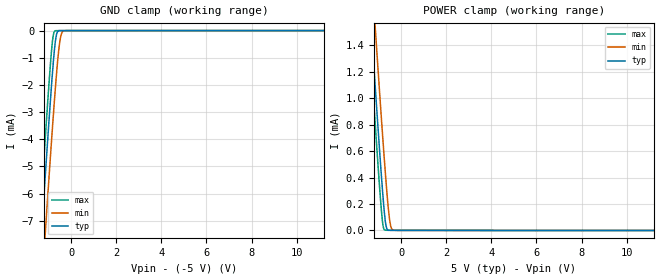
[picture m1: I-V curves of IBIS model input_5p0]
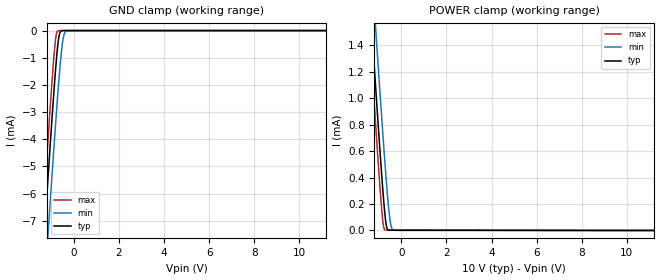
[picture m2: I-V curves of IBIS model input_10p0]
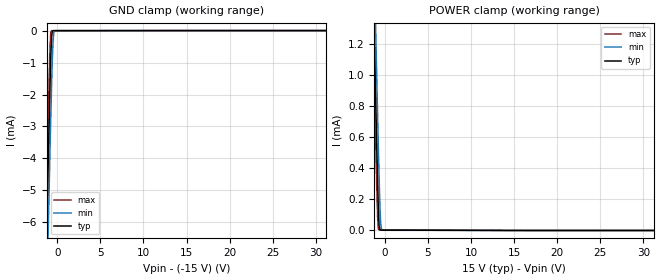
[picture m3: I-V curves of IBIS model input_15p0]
|Texas Instruments Incorporated
|TMUX6113, 36-V, Low-Capacitance, Low-Leakage-Current, Precision,
|Quad SPST Switches (Dual Open + Dual Closed)
[IBIS Ver]   4.1
[File name]   tmux6113.ibs
[Date]   10/26/2018
[File Rev]   1.0
[Source]
| Texas Instruments Incorporated.
| Analog-eLab Design Center, HPA
| 12500 TI Blvd
| Dallas, TX -75243
[Notes]   Revision History:
| Rev 1.0: 10/26/2018
| - Initial version of the model
| - Model generated from simulations in SPECTRE
| - Model names with a trailing _5p0 contain the model for 5.0V operation.
|   Model names with a trailing _10p0 contain the model for 10.0V operation.
|   Model names with a trailing _15p0 contain the model for 15.0V operation.
|   Model names with a trailing _33p0 contain the model for 33.0V operation.
| - C_comp although listed in numerical order of value are
|   obtained from varying PVT conditions. For PVT conditions for
|   each specific value refer the buffer description under
|   respective [Model]. IBIS model user is responsible for using
|   appropriate C_comp to simulate for Signal Integrity.
[Disclaimer]
| This model is designed as an aid for customers of Texas Instruments.
| TI and its licensors and suppliers make no warranties, either expressed
| or implied, with respect to this  model, including the warranties of
| merchantability or fitness for a particular purpose. The model is
| provided solely on an "as is" basis. The entire risk as to its quality
| and performance is with the customer.
| This model is subject to change without notice. Texas Instruments
| Incorporated is not responsible for updating this model.
[Copyright]
(C) Copyright 2018 Texas Instruments Incorporated.All rights reserved.
|  Component TMUX6113PW 16-Pin TSSOP -PW package
|  Part # TMUX6113PW
[Component]   TMUX6113PW
[Manufacturer]   TI
[Package]   |16 TSSOP -PW package
|   typ   min   max
R_pkg   0.05   0.04   0.06
L_pkg   1.0nH   0.8nH   1.2nH
C_pkg   0.2pF   0.16pF   0.24pF
[Pin] signal_name  model_name   R_pin   L_pin   C_pin
1   SEL1   INPUT   NA   NA   NA
2   D1   NC   NA   NA   NA
3   S1   NC   NA   NA   NA
4   VSS   POWER   NA   NA   NA
5   GND   GND   NA   NA   NA
6   S4   NC   NA   NA   NA
7   D4   NC   NA   NA   NA
8   SEL4   INPUT   NA   NA   NA
9   SEL3   INPUT   NA   NA   NA
10   D3   NC   NA   NA   NA
11   S3   NC   NA   NA   NA
12   NC   NC   NA   NA   NA
13   VDD   POWER   NA   NA   NA
14   S2   NC   NA   NA   NA
15   D2   NC   NA   NA   NA
16   SEL2   INPUT   NA   NA   NA
|  Component TMUX6113RTE 16-Pin WQFN -RTE package
|  Part # TMUX6113RTE
[Component]   TMUX6113RTE
[Manufacturer]   TI
[Package]   |16 WQFN -RTE package
|   typ   min   max
R_pkg   0.05   0.04   0.06
L_pkg   1.0nH   0.8nH   1.2nH
C_pkg   0.2pF   0.16pF   0.24pF
[Pin] signal_name  model_name   R_pin   L_pin   C_pin
1   S1   NC   NA   NA   NA
2   VSS   POWER   NA   NA   NA
3   GND   GND   NA   NA   NA
4   S4   NC   NA   NA   NA
5   D4   NC   NA   NA   NA
6   SEL4   INPUT   NA   NA   NA
7   SEL3   INPUT   NA   NA   NA
8   D3   NC   NA   NA   NA
9   S3   NC   NA   NA   NA
10   NC   NC   NA   NA   NA
11   VDD   POWER   NA   NA   NA
12   S2   NC   NA   NA   NA
13   D2   NC   NA   NA   NA
14   SEL2   INPUT   NA   NA   NA
15   SEL1   INPUT   NA   NA   NA
16   D1   NC   NA   NA   NA
|   Model Selectors
[Model Selector] INPUT
input_5p0   5V   digital Input
input_10p0   10V   digital Input
input_15p0   15V   digital Input
input_33p0   33V   digital Input
| Models and submodels in the file (4): input_5p0 (Input), input_10p0 (Input), input_15p0 (Input), input_33p0 (Input)
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|   input_5p0 Model
[Model]   input_5p0
Model_type   Input
Vinl = 2
Vinh = 0.8
|   typ   min   max
C_comp   0.358pF   0.356pF   0.361pF
| Where Nom  PVT is Nominal Process, 10V, 25C
|   Fast PVT is Strong Process,  11V, -40C
|   Slow PVT is Weak Process,   09V, 125C
[Voltage Range]   10   9   11
|Junction Temperature
[Temperature Range]   27   125   -40
[Power Clamp Reference]   5   4.5   5.5
[GND Clamp Reference]   -5   -4.5   -5.5
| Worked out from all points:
|   GND clamp passes 1 mA (typ) near -0.77 V on its own axis
|   POWER clamp passes 1 mA (typ) near -1.11 V on its own axis
[GND Clamp]
|   Voltage   I(typ)   I(min)   I(max)
-10V      -122.7mA   -124.2mA   -121.9mA
-1.42V    -8.845mA   -10.94mA   -7.472mA
-1.27V    -6.929mA   -9.033mA   -5.544mA
-1.15V    -5.415mA   -7.523mA   -4.026mA
-970mV    -3.204mA   -5.296mA   -1.838mA
-850mV    -1.816mA   -3.855mA   -580.2uA
-790mV    -1.182mA   -3.156mA   -171.6uA
-700mV    -414.1uA   -2.152mA   -7.066uA
-610mV    -53.99uA   -1.244mA   -1.599uA
-490mV    -1.686uA   -354.5uA   -1.486uA
-310mV    -846.9nA   -6.833uA   -1.443uA
20V       0A         0A         0A
[POWER Clamp]
|   Voltage   I(typ)   I(min)   I(max)
-10V      24.94mA    25.34mA    24.69mA
-1.42V    1.795mA    2.242mA    1.511mA
-1.3V     1.483mA    1.93mA     1.197mA
-1.12V    1.02mA     1.467mA    735uA
-850mV    360.2uA    790.9uA    107.9uA
-790mV    229.4uA    646.8uA    26.21uA
-700mV    70.11uA    438.8uA    2.029uA
-640mV    16.14uA    308.9uA    1.563uA
-520mV    1.094uA    94.98uA    1.508uA
-430mV    885.2nA    17.06uA    1.485uA
-340mV    864.3nA    1.97uA     1.463uA
20V       0A         0A         0A
|   input_10p0 Model
[Model]   input_10p0
Model_type   Input
Vinl = 2
Vinh = 0.8
|   typ   min   max
C_comp   0.366pF   0.363pF   0.370pF
| Where Nom  PVT is Nominal Process, 10V, 25C
|   Fast PVT is Strong Process,  11V, -40C
|   Slow PVT is Weak Process,   09V, 125C
[Voltage Range]   10   9   11
|Junction Temperature
[Temperature Range]   27   125   -40
[Power Clamp Reference]   10   9   11
[GND Clamp Reference]   0   0   0
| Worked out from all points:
|   GND clamp passes 1 mA (typ) near -0.77 V on its own axis
|   POWER clamp passes 1 mA (typ) near -1.11 V on its own axis
[GND Clamp]
|   Voltage   I(typ)   I(min)   I(max)
-10V      -122.7mA   -124.2mA   -121.9mA
-1.42V    -8.845mA   -10.94mA   -7.472mA
-1.27V    -6.929mA   -9.033mA   -5.544mA
-1.15V    -5.415mA   -7.522mA   -4.025mA
-970mV    -3.204mA   -5.296mA   -1.838mA
-850mV    -1.816mA   -3.855mA   -579.6uA
-790mV    -1.182mA   -3.156mA   -170.8uA
-700mV    -413.6uA   -2.152mA   -5.772uA
-610mV    -53.35uA   -1.244mA   -201.1nA
-490mV    -861.9nA   -354.2uA   -85nA
-310mV    -14.25nA   -6.398uA   -42.25nA
20V       0A         0A         0A
[POWER Clamp]
|   Voltage   I(typ)   I(min)   I(max)
-10V      24.94mA    25.34mA    24.69mA
-1.42V    1.796mA    2.243mA    1.512mA
-1.3V     1.484mA    1.931mA    1.199mA
-1.12V    1.021mA    1.467mA    736.4uA
-850mV    361uA      791.3uA    109.3uA
-790mV    230.2uA    647.2uA    27.61uA
-700mV    70.94uA    439.2uA    3.429uA
-640mV    16.97uA    309.4uA    2.964uA
-520mV    1.927uA    95.44uA    2.909uA
-430mV    1.718uA    17.52uA    2.886uA
-340mV    1.697uA    2.425uA    2.863uA
20V       0A         0A         0A
|   input_15p0 Model
[Model]   input_15p0
Model_type   Input
Vinl = 2
Vinh = 0.8
|   typ   min   max
C_comp   0.331pF   0.328pF   0.334pF
| Where Nom  PVT is Nominal Process, 30V, 25C
|   Fast PVT is Strong Process,  33V, -40C
|   Slow PVT is Weak Process,   27V, 125C
[Voltage Range]   30   27   33
|Junction Temperature
[Temperature Range]   27   125   -40
[Power Clamp Reference]   15   13.5   16.5
[GND Clamp Reference]   -15   -13.5   -16.5
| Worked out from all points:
|   GND clamp passes 1 mA (typ) near -0.77 V on its own axis
|   POWER clamp passes 1 mA (typ) near -1.11 V on its own axis
[GND Clamp]
|   Voltage   I(typ)   I(min)   I(max)
-30V      -408mA     -425.8mA   -391.2mA
-1.38V    -8.333mA   -10.43mA   -6.957mA
-1.29V    -7.184mA   -9.286mA   -5.801mA
-1.2V     -6.044mA   -8.15mA    -4.656mA
-1.11V    -4.917mA   -7.023mA   -3.528mA
-1.02V    -3.809mA   -5.909mA   -2.428mA
-840mV    -1.707mA   -3.737mA   -497.3uA
-750mV    -804.6uA   -2.702mA   -49.55uA
-660mV    -197.4uA   -1.733mA   -5.082uA
-480mV    -3.007uA   -305.9uA   -4.207uA
-210mV    -2.425uA   -1.669uA   -4.152uA
60V       0A         0A         0A
[POWER Clamp]
|   Voltage   I(typ)   I(min)   I(max)
-30V      151.4mA    209.2mA    94.31mA
-1.38V    1.693mA    2.139mA    1.409mA
-1.29V    1.458mA    1.905mA    1.174mA
-1.2V     1.226mA    1.673mA    941.7uA
-1.11V    996.3uA    1.442mA    712.5uA
-1.02V    770uA      1.214mA    488.8uA
-840mV    339.3uA    767.5uA    93.31uA
-750mV    152.4uA    553.7uA    9.343uA
-660mV    29.88uA    352uA      4.367uA
-480mV    2.552uA    50.19uA    4.256uA
-300mV    2.481uA    1.811uA    4.212uA
60V       0A         0A         0A
